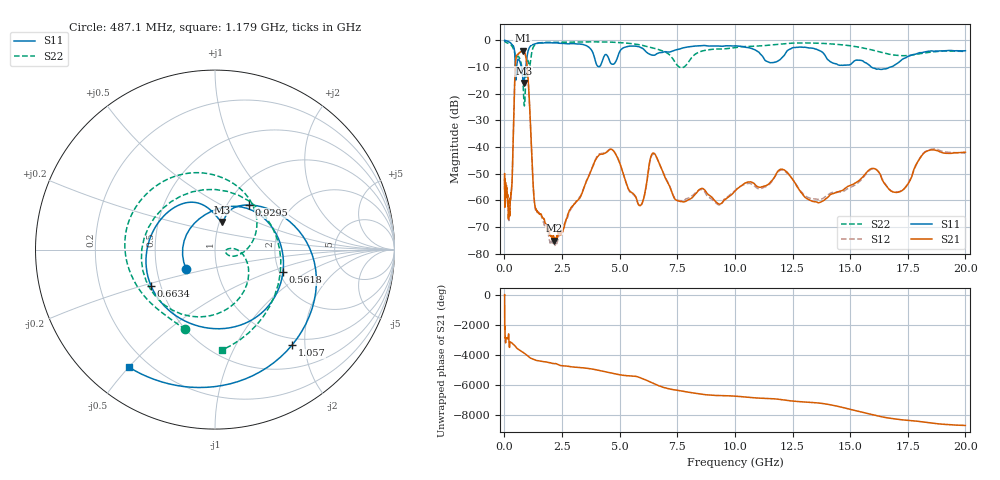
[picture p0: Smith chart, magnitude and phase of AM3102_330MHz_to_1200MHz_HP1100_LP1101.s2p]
! Date/Time: Tue, Sep 11, 2018 5:21 PM
! Network Analyzer: Agilent Technologies E8362B Rev: A.07.50.63
! Sweep from 0.010 to 20.000 GHz, 1601 Points, Sweep Type: LOG
! Power Supply: 4.949 V, 0.001 A
# Hz S DB R 50
!freq MagS11 AngS11 MagS21 AngS21 MagS12 AngS12 MagS22 AngS22
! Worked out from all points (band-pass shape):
!   1601 points, 10 MHz to 20 GHz, reference 50 ohm
!   highest |S21| = -3.90 dB at 798.4 MHz (marker M1); lowest = -75.1 dB at 2.155 GHz (marker M2)
!   |S21| within 3 dB of the highest: 496 MHz to 944.3 MHz (448.2 MHz wide, 62.2 % of centre)
!   lowest |S11| = -16.0 dB at 837.2 MHz (marker M3), VSWR 1.38, Z = 51.4 + j16.3 ohm
!   |S11| at or under -10 dB: 471.3 MHz to 532.1 MHz (60.74 MHz wide, 12.1 % of centre); 740.3 MHz to 930.4 MHz (190.1 MHz wide, 22.8 % of centre); 15.91 GHz to 16.76 GHz (846.8 MHz wide, 5.18 % of centre)
!   |S22| runs from -24.6 to -0.2 dB; largest |S21 - S12| = 0.0098
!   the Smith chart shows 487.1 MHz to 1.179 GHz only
!   S11 on the Smith chart (normalised r, x): 487.1 MHz: 0.71, -0.16; 561.8 MHz: 2.09, -0.63; 663.4 MHz: 0.44, -0.21; 929.5 MHz: 1.26, +0.69; 1.057 GHz: 0.87, -1.75; 1.179 GHz: 0.13, -0.50
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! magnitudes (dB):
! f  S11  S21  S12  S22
! 10 MHz  -0.1  -50.1  -52.0  -0.2
! 35.55 MHz  -0.1  -59.3  -61.0  -0.5
! 126.4 MHz  -0.3  -57.9  -58.3  -1.0
! 316.2 MHz  -1.5  -54.8  -55.4  -2.0
! 447.2 MHz  -4.6  -15.7  -15.7  -4.6
! 487.1 MHz  -14.2  -7.7  -7.7  -6.5
! 561.8 MHz  -8.0  -5.5  -5.4  -6.1
! 663.4 MHz  -7.8  -4.6  -4.7  -6.8
! 798.4 MHz  -14.1  -3.9  -4.0  -14.4
! 837.2 MHz  -16.0  -4.1  -4.1  -21.2
! 929.5 MHz  -10.1  -6.2  -6.2  -14.2
! 1.057 GHz  -3.3  -18.3  -18.3  -8.8
! 1.179 GHz  -1.8  -41.3  -41.3  -5.0
! 1.327 GHz  -1.3  -62.0  -62.9  -1.7
! 1.59 GHz  -1.0  -65.3  -65.3  -0.9
! 2.155 GHz  -1.0  -75.1  -75.7  -0.7
! 4.171 GHz  -9.4  -42.8  -42.5  -0.6
! 5.652 GHz  -2.2  -58.1  -58.4  -1.4
! 6.518 GHz  -5.6  -42.5  -42.9  -3.0
! 7.625 GHz  -3.2  -60.4  -60.1  -10.2
! 13.61 GHz  -3.7  -60.9  -59.7  -1.1
! 20 GHz  -3.9  -42.0  -42.4  -4.2
